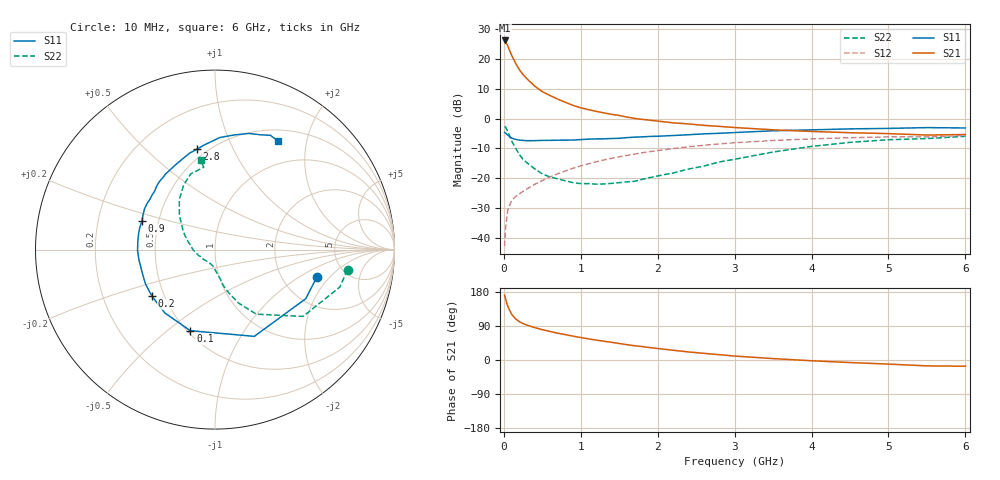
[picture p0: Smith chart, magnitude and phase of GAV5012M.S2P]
! Infineon Technologies  Discrete & RF Semiconductors
! BF775
! Si NPN RF Bipolar Junction Transistor in SOT23
! VCE = 0.5 V  IC = 12 mA
! Common Emitter S-Parameters:  May  1996
# GHz  S  MA  R  50
!  f  S11  S21  S12  S22
! GHz  MAG  ANG  MAG  ANG  MAG  ANG  MAG  ANG
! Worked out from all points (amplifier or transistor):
!   36 points, 10 MHz to 6 GHz, reference 50 ohm
!   highest |S21| = 26.3 dB at 10 MHz (marker M1)
!   |S21| within 3 dB of that: start of sweep to 69.26 MHz
!   unconditionally stable (mu >= 1): start of sweep to 10.28 MHz; 172 MHz to end of sweep
!   at 250 MHz: K = 1.26, MAG = 16.6 dB, |S12| = -24.4 dB
!   at 1.4 GHz: K = 1.66, MAG = 2.7 dB, |S12| = -13.3 dB
!   at 6 GHz: K = 1.17, MAG = -2.3 dB, |S12| = -5.6 dB
!   S11 on the Smith chart (normalised r, x): 10 MHz: 3.11, -1.45; 100 MHz: 0.52, -0.60; 200 MHz: 0.43, -0.27; 900 MHz: 0.40, +0.16; 2.8 GHz: 0.44, +0.73; 6 GHz: 0.65, +1.54
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0.01  0.5875 -15.1  20.64 171.2  0.0072 79.1  0.7469 -8.7
0.02  0.575 -28.4  19.99 162.9  0.0134 75.8  0.726 -16.7
0.05  0.5307 -65.6  16.79 142.1  0.0288 61.6  0.6157 -37.2
0.1  0.4723 -106.9  11.71 121.1  0.0418 49.7  0.427 -57.4
0.15  0.4502 -128.5  8.683 109.1  0.049 47.7  0.3247 -66.3
0.2  0.4368 -143.6  6.713 101.5  0.0543 48.6  0.252 -72.5
0.25  0.4318 -153.7  5.504 96.2  0.0601 49.9  0.2065 -76.9
0.3  0.4265 -160.4  4.698 92.2  0.0661 52.0  0.1818 -78.3
0.4  0.4275 -172.2  3.533 85.6  0.0786 54.4  0.1442 -82.9
0.5  0.4314 -179.2  2.851 80.1  0.0913 56.6  0.1178 -88.3
0.6  0.4322 174.4  2.454 75.4  0.1046 57.3  0.1049 -91.8
0.7  0.4349 168.4  2.135 70.8  0.1185 58.0  0.0976 -94.4
0.9  0.4369 158.8  1.673 63.0  0.1471 57.7  0.0841 -105.5
1.1  0.453 150.3  1.419 55.9  0.1748 56.2  0.0811 -118.9
1.3  0.4582 142.6  1.252 49.5  0.2026 54.0  0.0799 -130.7
1.7  0.4897 129.1  1.009 37.6  0.2543 49.1  0.0885 -153.6
2.2  0.521 115.0  0.852 25.8  0.3146 41.8  0.1223 -179.7
2.8  0.5678 100.3  0.743 14.0  0.3767 32.5  0.1873 154.2
3.5  0.6256 87.4  0.65 3.7  0.43 21.7  0.2754 136.1
4.5  0.6739 73.8  0.581 -6.7  0.4792 8.0  0.4 115.9
5.5  0.7076 64.1  0.531 -15.5  0.4934 -4.3  0.4629 97.8
6  0.6981 59.7  0.542 -16.4  0.5228 -7.9  0.5057 99.1
